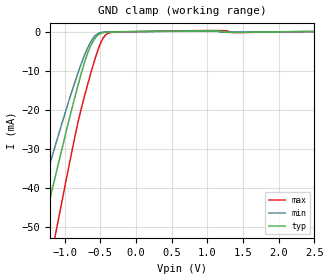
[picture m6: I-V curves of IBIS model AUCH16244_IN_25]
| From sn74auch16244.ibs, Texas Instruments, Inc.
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[Model]   AUCH16244_IN_25
Model_type  Input
Vinl=0.7
Vinh=1.7
| variable   typ   min   max
C_comp   3.36pF   2.47pF   3.89pF
[Temperature Range]   40   100   -40
| Ambient temperature   25   85   -40
[Voltage range]   2.5   2.3   2.7
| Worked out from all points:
|   GND clamp passes 1 mA (typ) near -0.54 V on its own axis
[GND Clamp]
| AUCH16244_IN_25
|   Voltage   I(typ)   I(min)   I(max)
-3.6V     -232.7mA   -194.4mA   -280.6mA
-1.525V   -67.94mA   -54.42mA   -89.19mA
-1.465V   -63.22mA   -50.53mA   -83.59mA
-1.3V     -50.32mA   -39.94mA   -68.18mA
-1.11V    -35.67mA   -28.03mA   -50.42mA
-840mV    -15.73mA   -12.13mA   -25.66mA
-720mV    -7.899mA   -6.049mA   -16.5mA
-625mV    -3.315mA   -2.379mA   -10.19mA
-520mV    -760.3uA   -417uA     -4.107mA
-425mV    -164.1uA   -95.31uA   -878.5uA
-315mV    -74.11uA   -47.66uA   -146.2uA
2.5V      355.7pA    563.3nA    -12.78nA
